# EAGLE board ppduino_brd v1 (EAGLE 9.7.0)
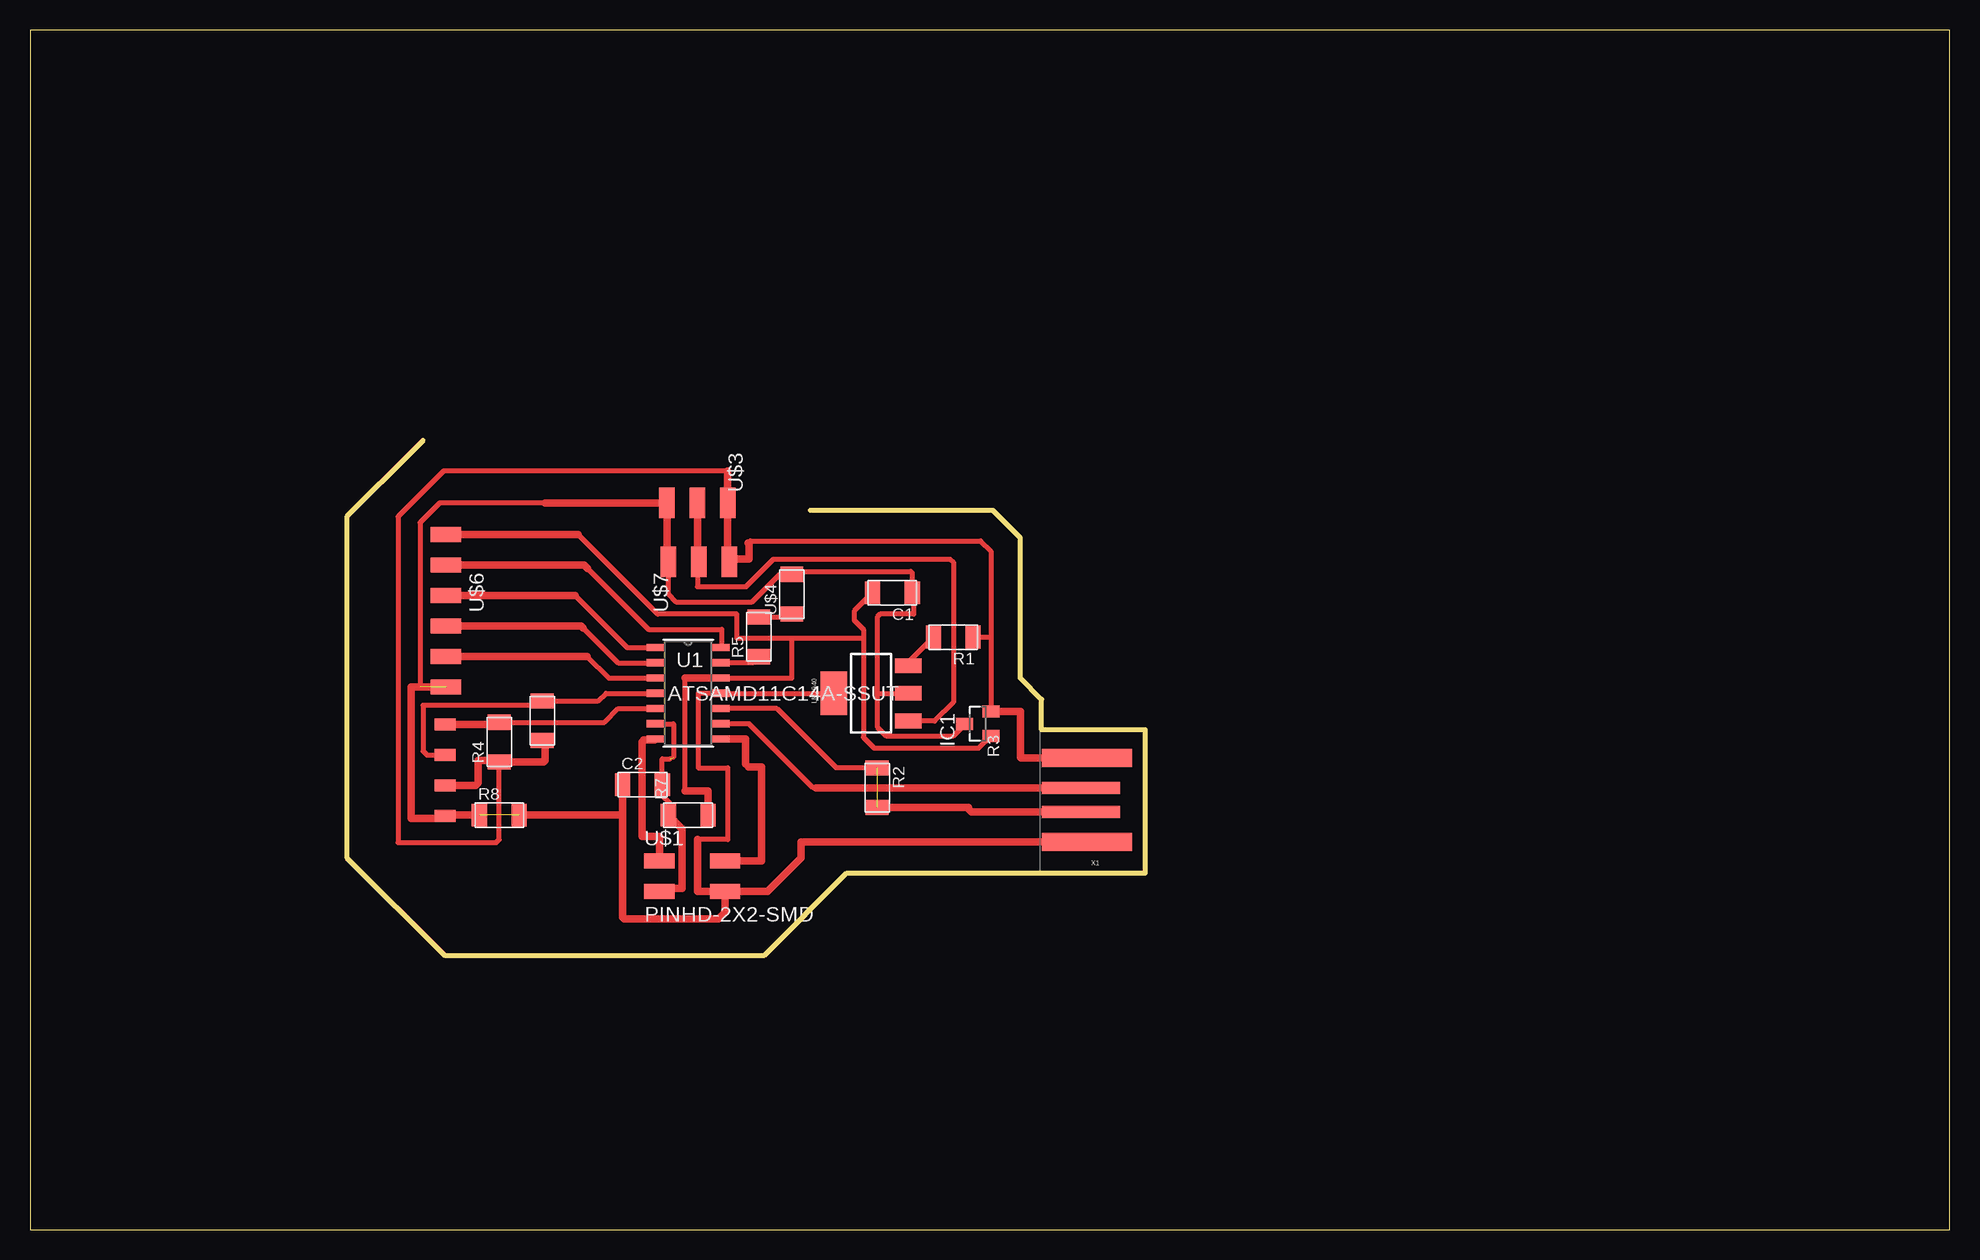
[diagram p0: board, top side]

Size 160 x 100 mm. Coordinates in mm from the lower left corner, seen from the top.
Outline: 32.77,65.79 32,65.02 26.42,59.44 26.42,30.99 34.54,22.86 61.21,22.86 68.07,29.72 92.96,29.72 92.96,41.66 84.33,41.66 84.33,44.2 82.55,45.97 82.55,57.66 80.26,59.94 65.02,59.94
Outline: 0,0 160,0 160,100 0,100 0,0
Copper layers (1*16): Top / Bottom
Stack-up Default Layer Stack: Top User Defined 0.035mm / Dielectric-1 User Defined 1.5mm / Bottom User Defined 0.035mm
Design rules "default *": minimum track width 16mil, minimum drill 0.35mm, track to track 6mil, track to pad 6mil, pad to pad 6mil, via to via 6mil, smd to smd 6mil, copper to edge 40mil, drill to drill 6mil, minimum pad ring 10mil, minimum via ring 8mil, stop-mask expansion 4mil, vias tented up to drill 0mil, thermal gap 10mil

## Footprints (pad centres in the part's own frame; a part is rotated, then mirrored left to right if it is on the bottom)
C1206FAB = smd 1.27 x 1.905: 1 -1.651,0; 2 1.651,0
SOT23 = smd 1 x 1.4: 1 -1.001,-1.1; 2 1.014,-1.1; 3 0,1.1
1X04SMD/90 = smd 1.016 x 1.778: 1 -1.27,-5.08; 2 1.27,-5.08; 3 3.81,-5.08; 4 6.35,-5.08
SOT223 = smd 1.219 x 2.235: 1 -2.311,-3.099; 2 0,-3.099; 3 2.311,-3.099 | smd 3.6 x 2.2: 4 0,3.099
R1206FAB = smd 1.27 x 1.905: 1 -1.651,0; 2 1.651,0
SOIC14_SL_MCH = smd 1.5 x 0.6: 1 -2.7,3.81; 2 -2.7,2.54; 3 -2.7,1.27; 4 -2.7,0; 5 -2.7,-1.27; 6 -2.7,-2.54; 7 -2.7,-3.81; 8 2.7,-3.81; 9 2.7,-2.54; 10 2.7,-1.27; 11 2.7,0; 12 2.7,1.27; 13 2.7,2.54; 14 2.7,3.81
2X02SMD = smd 2.54 x 1.27: 1 -2.54,1.27; 2 2.92,1.27; 3 -2.54,-1.27; 4 2.92,-1.27
SPDTSWITCH = smd 2.54 x 1.27: 1 0.38,2.54; 2 0.38,0; 3 0.38,-2.54
LED1206FAB = smd 1.27 x 1.905: 1 -1.651,0; 2 1.651,0
1X06SMD = smd 2.54 x 1.27: 1 0,6.35; 2 0,3.81; 3 0,1.27; 4 0,-1.27; 5 0,-3.81; 6 0,-6.35
USB-A-PCB = smd 7.5 x 1.5: 5V -0.2,-3.5; GND -0.2,3.5 | smd 6.5 x 1: USB_M 0.3,-1; USB_P 0.3,1

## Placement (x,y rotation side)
C1  1uF  [C1206FAB]  71.88,53.09 180 top
C2  1uF  [C1206FAB]  51.05,37.08 0 top
IC1  [SOT23]  78.99,42.16 90 top
JP3  [1X04SMD/90]  29.53,35.74 90 top
LM2940  VR_REGULATOR_SOT223  [SOT223]  70.1,44.7 90 top
R1  [R1206FAB]  76.96,49.39 180 top
R2  0  [R1206FAB]  70.61,36.83 270 top
R3  4.99K  [R1206FAB]  42.7,42.42 90 top
R4  4.99K  [R1206FAB]  39.12,40.64 90 top
R5  1K  [R1206FAB]  60.75,49.41 90 top
R7  10K  [R1206FAB]  54.86,34.54 0 top
R8  0  [R1206FAB]  39.12,34.54 0 top
U1  ATSAMD11C14A-SSUT  [SOIC14_SL_MCH]  54.86,44.7 0 top
U$1  PINHD-2X2-SMD  [2X02SMD]  55.02,29.46 0 top
U$3  SPDTSWITCH  [SPDTSWITCH]  55.63,60.96 270 top
U$4  LEDFAB1206  [LED1206FAB]  63.5,52.97 90 top
U$6  CONN_06_FTDI-SMD-HEADER  [1X06SMD]  34.67,51.59 180 top
U$7  SPDTSWITCH  [SPDTSWITCH]  55.75,55.28 90 top
X1  CONN_USBPCB  [USB-A-PCB]  87.88,35.81 180 top

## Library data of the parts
C1 C2 IC1 LM2940 R1-R5 R7 R8 U$1 U$3 U$4 U$6 U$7 X1 = fab
JP3 = pinhead-2
U1 = samd11c; BUILT_BY: EMA_Molly; COPYRIGHT: Copyright (C) 2018 Accelerated Designs. All rights reserved; MANUFACTURER_PART_NUMBER: ATSAMD11C14A-SSUT; SOURCELIBRARY: Microchip_2019-08-23_25; VENDOR: Microchip

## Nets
2: R5.1 U1.13
4: U1.14 U$6.5
5: U1.1 U$6.4
5V: IC1.2 JP3.2 R1.1 R3.1 R4.1 U$3.1 U$7.3 X1.5V
5VA: LM2940.3 R1.2
8: U1.2 U$6.3
9: U1.3 U$6.2
24-: U1.9 X1.USB_M
25+: R2.1 R2.2 U1.10 X1.USB_P
CLK: U1.7 U$1.1
DIO: U1.8 U$1.2
GND: C1.1 C2.1 IC1.3 JP3.1 LM2940.2 LM2940.4 R8.1 R8.2 U1.11 U$1.4 U$3.3 U$4.2 U$6.1 U$7.1 X1.GND
N$5: R5.2 U$4.1
RST: C2.2 R7.1 U1.6 U$1.3
SCL: JP3.4 R4.2 U1.5
SDA: JP3.3 R3.2 U1.4
VD0: LM2940.1 U$3.2 U$7.2
VDD: C1.2 IC1.1 R7.2 U1.12 U$6.6

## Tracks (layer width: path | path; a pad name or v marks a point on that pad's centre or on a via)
2
  Top 0.406: U1.13 60.24,47.24 R5.1
4
  Top 0.406: 46.48,55.12 51.56,50.04 57.66,50.04 57.66,48.61 U1.14
  Top 0.61: U$6.5 46.2,55.4 46.48,55.12
5
  Top 0.406: 45.44,52.86 49.78,48.51 U1.1
  Top 0.61: U$6.4 45.44,52.86
5V
  Top 0.406: 58.17,59.94 U$3.1 | 87.63,39.77 X1.5V | IC1.2 80.09,49.39 | 82.55,39.37 82.61,39.31 | 59.86,57.23 60.04,57.4 79.25,57.4 80.09,56.56 80.09,49.39 | R4.1 39.12,32.51 38.86,32.26 30.68,32.26 30.68,59.44 34.49,63.25 58.17,63.25 | R1.1 80.09,49.39
  Top 0.61: 58.17,59.94 58.17,55.78 U$7.3 58.52,55.88 59.94,55.88 59.94,57.15 59.86,57.23 | JP3.2 37.14,37.01 37.34,37.21 37.34,39.12 38.99,39.12 R4.1 42.8,38.99 42.93,39.12 42.93,40.54 R3.1 | U$3.1 58.17,63.25 | IC1.2 82.55,43.18 | 82.55,43.18 | 82.55,43.18 82.55,39.37 | X1.5V 82.61,39.31
5VA
  Top 0.406: LM2940.3 73.2,47.28 R1.2
8
  Top 0.406: 46.1,50.16 49.02,47.24 U1.2
  Top 0.61: U$6.3 45.95,50.32 46.1,50.16
9
  Top 0.406: 46.46,47.78 48.26,45.97 U1.3
  Top 0.61: U$6.2 46.46,47.78
24-
  Top 0.406: U1.9 59.94,42.16 65.28,36.83 65.53,36.83
  Top 0.61: X1.USB_M 65.55,36.81 65.53,36.83
25+  (1 unrouted)
  Top 0.406: R2.1 67.21,38.48 62.26,43.43 U1.10
  Top 0.61: R2.2 78.23,35.18 78.23,35.05 78.49,34.8 78.5,34.81 X1.USB_P
CLK
  Top 0.406: 51.03,40.66 51.16,40.8
  Top 0.61: 51.03,40.66 51.03,32.77 52.48,32.77 U$1.1 | U1.7 52.07,40.8 51.16,40.8
DIO
  Top 0.508: 59.64,38.81 59.9,38.56
  Top 0.61: U$1.2 60.96,30.73 60.96,38.56 59.9,38.56 | U1.8 59.64,40.89 59.64,38.81
GND  (2 unrouted)
  Top 0.406: LM2940.4 U1.11 55.69,44.7 55.69,38.48 58.17,38.48 58.17,32.51 55.63,32.51 | 53.09,60.2 U$3.3 | U$7.1 53.21,52.96 53.85,52.32 60.2,52.32 62.49,54.62 U$4.2 63.75,54.86 73.41,54.86 73.53,54.74 C1.1 73.66,52.96 73.66,51.31 70.87,51.31 70.61,51.05 70.61,44.7 | 42.93,60.58 34.16,60.58 32.51,58.93 32.51,45.21 | 70.61,44.7 LM2940.2 | 70.61,44.7 70.61,41.91 71.37,41.15 76.96,41.15 77.89,42.08 IC1.3
  Top 0.508: 64.52,32.31 64.26,32.31
  Top 0.61: U$1.4 57.94,26.44 57.4,25.91 49.53,25.91 49.4,26.04 49.4,34.54 | C2.1 49.4,34.54 | U$7.1 53.09,55.78 53.09,60.2 | R8.1 34.68,34.54 JP3.1 34.42,34.29 31.75,34.29 31.75,45.24 U$6.1 | R8.2 49.4,34.54 | U$1.4 55.63,28.19 55.63,32.51 | U$1.4 61.47,28.19 64.26,30.99 64.26,32.31 | U$3.3 42.93,60.58 | X1.GND 64.52,32.31
N$5
  Top 0.406: R5.2 63.25,51.06 U$4.1
RST  (1 unrouted)
  Top 0.406: 53.4,34.35 R7.1 53.34,34.67 53.34,35.56 52.7,36.2 C2.2 52.7,39.24 53.37,39.24 | U1.6 53.62,42.16 53.62,39.37
  Top 0.61: U$1.3 52.73,28.45 54.36,28.45 54.36,33.4 53.4,34.35
SCL
  Top 0.406: R4.2 47.88,42.29 49.02,43.43 U1.5
  Top 0.61: JP3.4 38.92,42.09 R4.2
SDA
  Top 0.406: U1.4 48.01,44.7 47.37,44.07 R3.2 42.31,43.69 32.77,43.69 32.77,39.88 33.09,39.55 JP3.3
VD0
  Top 0.406: 55.63,59.94 U$3.2 | 55.63,55.78 55.63,53.59 59.69,53.59 61.98,55.88 76.71,55.88 76.96,55.63 76.96,43.94 75.41,42.39 LM2940.1
  Top 0.61: U$7.2 55.63,55.78 55.63,59.94
VDD
  Top 0.406: U1.12 63.5,45.97 63.5,49.28 | 70.23,52.7 C1.2 68.71,51.56 68.71,50.8 69.47,50.04 69.47,49.28 | 45.7,57.94 52.32,51.31 58.93,51.31 58.93,49.28 63.5,49.28 | 69.47,49.28 69.47,41.02 70.36,40.13 79.06,40.13 IC1.1 | 69.47,49.28 63.5,49.28 | 54.61,36.58 54.61,45.97
  Top 0.61: U1.12 54.61,45.97 | U$6.6 45.7,57.94 | R7.2 56.52,36.58 54.61,36.58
